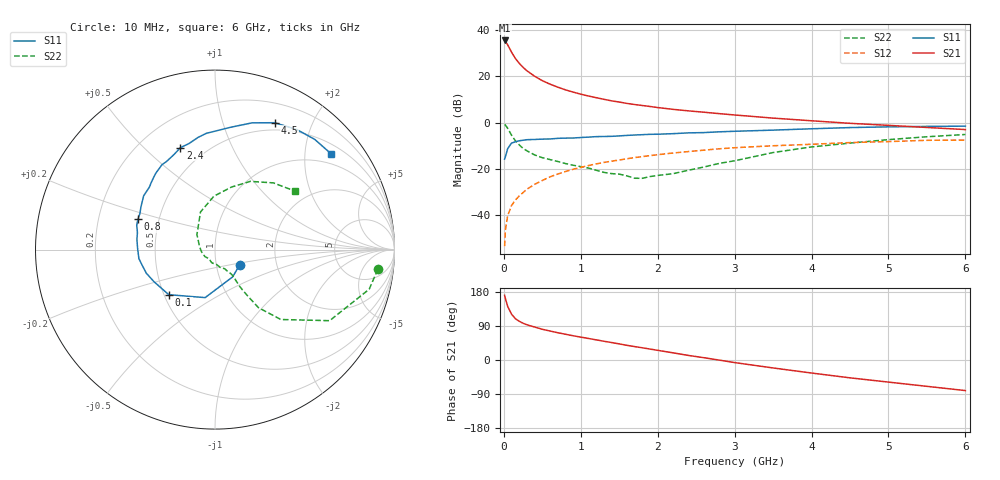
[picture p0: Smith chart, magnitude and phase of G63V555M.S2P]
! SIEMENS Small Signal Semiconductors
! BFG193
! Si NPN RF Bipolar Junction Transistor in SOT223
! VCE = 3.5 V  IC = 55 mA
! Common Emitter S-Parameters:  August  1996
# GHz  S  MA  R  50
!  f  S11  S21  S12  S22
! GHz  MAG  ANG  MAG  ANG  MAG  ANG  MAG  ANG
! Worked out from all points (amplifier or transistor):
!   36 points, 10 MHz to 6 GHz, reference 50 ohm
!   highest |S21| = 35.6 dB at 10 MHz (marker M1)
!   |S21| within 3 dB of that: start of sweep to 67.28 MHz
!   unconditionally stable (mu >= 1): 399.7 MHz to 2.361 GHz
!   at 250 MHz: K = 0.94, MSG = 27.1 dB, |S12| = -30.3 dB
!   at 1.4 GHz: K = 1.05, MAG = 11.7 dB, |S12| = -16.7 dB
!   at 6 GHz: K = 0.90, MSG = 2.3 dB, |S12| = -7.5 dB
!   S11 on the Smith chart (normalised r, x): 10 MHz: 1.30, -0.22; 100 MHz: 0.53, -0.31; 800 MHz: 0.38, +0.16; 2.4 GHz: 0.37, +0.65; 4.5 GHz: 0.41, +1.50; 6 GHz: 0.72, +2.60
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0.01  0.1619 -31.0  60.4 170.7  0.0021 89.9  0.9137 -6.9
0.02  0.1811 -57.2  58.12 162.5  0.0047 82.8  0.887 -14.4
0.05  0.2731 -101.6  48.43 141.1  0.0096 70.7  0.7516 -31.8
0.1  0.3598 -135.7  33.77 121.1  0.016 65.9  0.5351 -46.7
0.15  0.3842 -152.3  24.61 109.0  0.021 67.0  0.4039 -53.2
0.2  0.4045 -161.0  19.33 102.2  0.0257 69.1  0.3299 -54.5
0.25  0.415 -167.8  15.75 97.0  0.0305 69.3  0.2759 -55.7
0.3  0.4269 -173.2  13.3 92.9  0.0361 69.8  0.2451 -56.1
0.4  0.4314 179.1  10.13 87.0  0.046 70.3  0.1998 -55.9
0.5  0.4389 172.5  8.124 81.1  0.0557 68.9  0.1737 -55.6
0.6  0.4425 167.6  6.829 76.5  0.0668 67.8  0.1581 -57.0
0.7  0.4566 162.7  5.884 72.0  0.0767 66.7  0.144 -59.4
0.8  0.4615 158.6  5.141 68.0  0.0869 64.3  0.1299 -61.4
1.1  0.4851 146.8  3.773 56.8  0.1171 59.3  0.1037 -73.7
1.3  0.5003 139.9  3.203 49.5  0.1371 55.2  0.0835 -84.0
1.6  0.5285 130.2  2.607 38.7  0.1649 48.2  0.0701 -109.7
2.2  0.5766 113.4  1.939 18.9  0.2197 34.5  0.0782 -175.1
2.4  0.5998 108.7  1.798 12.0  0.2357 30.3  0.0929 162.4
3.5  0.6876 82.6  1.253 -21.0  0.3152 3.1  0.2247 111.1
4.5  0.7813 64.8  0.966 -47.1  0.3695 -16.9  0.3601 75.3
5.5  0.8281 47.9  0.785 -69.5  0.414 -40.3  0.4939 48.8
6  0.8385 39.6  0.707 -80.7  0.4195 -53.7  0.5532 36.0
